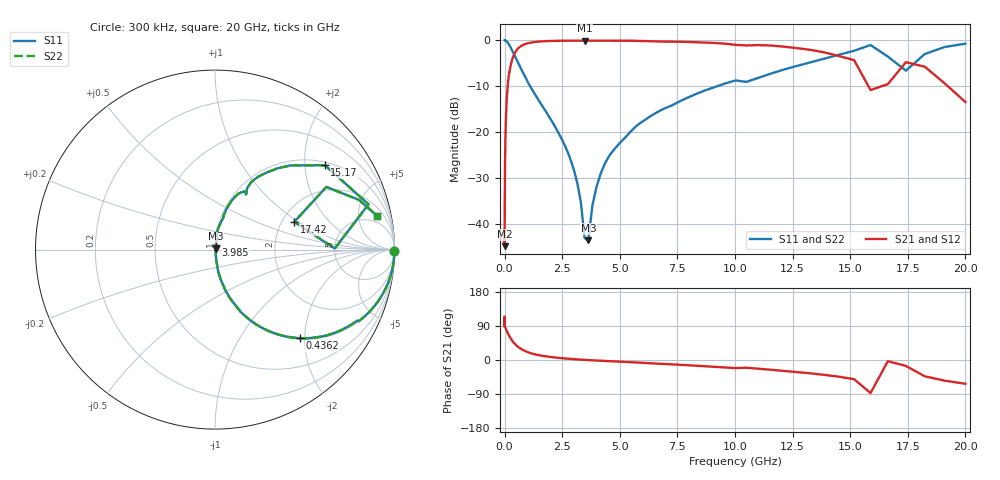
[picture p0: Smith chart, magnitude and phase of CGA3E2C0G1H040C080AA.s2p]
! S-parameter Generated by TDK Corporation
! Copyright(C) 2015 TDK Corporation.
! All Rights Reserved.
! TDK P/N: CGA3E2C0G1H040C080AA (Multilayer Ceramic Chip Capacitors)
! Property: C=4pF
! Size(LxWxT): 1.6x0.8x0.8mm, 0.063x0.031x0.031inches
! Model Type: s2p (Touchstone File Format Version 1.0)
! Frequency: DC=Yes Start=0.3MHz Stop=20000MHz 243points Log-sweep
! Note:
! Model Generated on Jun. 23, 2015
! Hash(MD5):
! Port Assignments:
!  1 ---| |--- 2
! Applicable Conditions:
!  Temperature = 25 degC
!  DC Bias Voltage = 0 V
!  Small Signal Operation
! Terms and conditions regarding TDK Simulation Models
! (1)This simulation model is being provided solely for informational purposes. Please refer to the specifications of the products in terms of detailed characteristics of such products.
! (2)In no event shall TDK Corporation of any of its subsidiaries be liable for any loss or damage arising, directly or indirectly,
!  From any information contained in this simulation model, including, but not limited to loss or damages arising from any inaccuracies, omissions or errors in connection with such information.
! (3)Any and all copyrights on this simulation model are owned by TDK Corporation.
!  Duplication or redistribution of this simulation model without prior written permission from TDK Corporation is prohibited.
! (4)This simulation model is subject to any modification or change without any prior notice.
! (5)Neither TDK Corporation nor any of its subsidiaries shall make any warranty, express or implied,
!  Including but not limited to the correctness, implied warranties of merchantability and fitness for a particular purpose with respect to this simulation models.
! (6)The use of this simulation model shall be deemed to have consented to the terms and conditions hereof.
# MHz S MA R 50
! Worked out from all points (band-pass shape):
!   242 points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, 300 kHz to 20 GHz, reference 50 ohm
!   highest |S21| = -0.04 dB at 3.471 GHz (marker M1); lowest = -44.9 dB at 994.4 kHz (marker M2)
!   |S21| within 3 dB of the highest: 414.8 MHz to 14.22 GHz (13.8 GHz wide, 189 % of centre)
!   lowest |S11| = -43.7 dB at 3.634 GHz (marker M3), VSWR 1.01, Z = 50.5 + j0.44 ohm
!   |S11| at or under -10 dB: 1.107 GHz to 9.225 GHz (8.118 GHz wide, 157 % of centre)
!   |S22| runs from -43.7 to 0.0 dB; largest |S21 - S12| = 3.3e-14
!   S11 on the Smith chart (normalised r, x): 300 kHz: open; 436.2 MHz: 1.02, -1.89; 3.985 GHz: 1.01, +0.05; 15.17 GHz: 1.09, +2.53; 17.42 GHz: 2.33, +0.92; 20 GHz: 3.31, +8.36
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0.3  1 -0.5  0.008553 89.5  0.008553 89.5  1 -0.5
0.9943584  0.9991 -0.3  0.005668 99.1  0.005668 99.1  0.9991 -0.3
1.985118  0.9995 -0.4  0.006587 93.7  0.006587 93.7  0.9995 -0.4
12.54397  0.9994 -1.8  0.03207 88.3  0.03207 88.3  0.9994 -1.8
79.26541  0.981 -11.2  0.1942 78.8  0.1942 78.8  0.981 -11.2
208.6529  0.8864 -26.5  0.4458 62.4  0.4458 62.4  0.8864 -26.5
436.1982  0.6824 -46.3  0.7229 43.0  0.7229 43.0  0.6824 -46.3
500.8786  0.6302 -50.4  0.7701 39.1  0.7701 39.1  0.6302 -50.4
1820.483  0.1631 -79.5  0.9833 9.4  0.9833 9.4  0.1631 -79.5
2632.185  0.06963 -83.0  0.9939 4.0  0.9939 4.0  0.06963 -83.0
3165.055  0.02705 -80.2  0.9957 1.5  0.9957 1.5  0.02705 -80.2
3470.673  0.006957 -54.2  0.9959 0.3  0.9959 0.3  0.006957 -54.2
3634.376  0.006538 41.8  0.9951 -0.3  0.9951 -0.3  0.006538 41.8
3985.312  0.025 78.6  0.9954 -1.4  0.9954 -1.4  0.025 78.6
5762.25  0.1191 81.6  0.9896 -6.8  0.9896 -6.8  0.1191 81.6
10985.48  0.388 62.4  0.8897 -22.8  0.8897 -22.8  0.388 62.4
15168.15  0.7716 37.6  0.6102 -50.5  0.6102 -50.5  0.7716 37.6
15883.6  0.8918 16.4  0.2874 -87.4  0.2874 -87.4  0.8918 16.4
16632.79  0.6672 0.5  0.3332 -3.2  0.3332 -3.2  0.6672 0.5
17417.32  0.4683 19.3  0.5792 -15.6  0.5792 -15.6  0.4683 19.3
18238.85  0.7115 29.4  0.5168 -43.1  0.5168 -43.1  0.7115 29.4
20000  0.922 11.8  0.2127 -62.7  0.2127 -62.7  0.922 11.8
